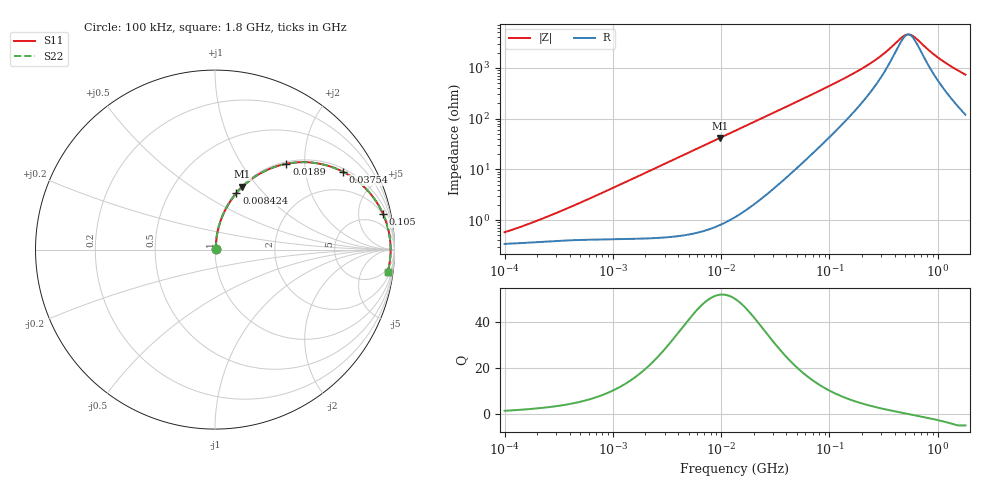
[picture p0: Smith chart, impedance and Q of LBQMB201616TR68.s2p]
! LBQMB201616TR68  S-PARAMETER MODEL  ( General Type )
! Model Generated by TAIYO YUDEN Corporation (http://www.ty-top.com)
! Version 1.0
! TAIYO YUDEN Control No. 191025NI43SB-FBB
! Copyright(c) 2019 TAIYO YUDEN CO.,LTD. All Rights Reserved.
! Product Description (link to TY-COMPAS)
! https://ds.yuden.co.jp/TYCOMPAS/or/detail?pn=LBQMB201616TR68J&u=M
! Products Name : Inductors
! Characteristics :
!  Inductance : 0.68 uH , SRF(min) : 270 MHz , DC Resistance(max) : 0.416 Ohm , Rated Current : 400 mA
!  Case Size : 2.0 x 1.6 / 0.079 x 0.063 [mm/inch] , Thickness : 1.6 / 0.063 [mm/inch]
!  (Conditions: Temperature = 25 degC , DC Bias Current/Voltage = 0A / 0V)
! External Node Assignments :
!  1  o---GGG---o  2
! GND o---------o GND
! Frequency Range : 0.1MHz  -  1800MHz  [ 402 STEP ]
# MHz S RI R 50
! Freq[MHz].  S11 Real  S11 Imag  S21 Real  S21 Imag  S12 Real  S12 Imag  S22 Real  S22 Imag
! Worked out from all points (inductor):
!   401 points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, 100 kHz to 1.8 GHz, reference 50 ohm
!   read as one part in series: L = 702 nH near 259.9 kHz
!   highest Q = 52 at 9.758 MHz (marker M1), where L = 680 nH
!   self-resonance near 535.3 MHz
!   S11 on the Smith chart (normalised r, x): 100 kHz: 1.01, +0.01; 8.424 MHz: 1.01, +0.72; 18.9 MHz: 1.04, +1.62; 37.54 MHz: 1.12, +3.22; 105 MHz: 1.96, +9.24; 1.8 GHz: 3, -15
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0.1  0.00341 0.00464  0.9966 -0.00464  0.9966 -0.00464  0.00341 0.00464
0.19855  0.00377 0.00892  0.9962 -0.00892  0.9962 -0.00892  0.00377 0.00892
0.516129  0.00456 0.0222  0.9954 -0.0222  0.9954 -0.0222  0.00456 0.0222
1.309209  0.00732 0.0554  0.9927 -0.0554  0.9927 -0.0554  0.00732 0.0554
2.66389  0.0171 0.1114  0.9829 -0.1114  0.9829 -0.1114  0.0171 0.1114
5.161158  0.0509 0.2082  0.9491 -0.2082  0.9491 -0.2082  0.0509 0.2082
8.423854  0.1195 0.3147  0.8805 -0.3147  0.8805 -0.3147  0.1195 0.3147
9.75753  0.1529 0.3504  0.8471 -0.3504  0.8471 -0.3504  0.1529 0.3504
13.41641  0.2518 0.4242  0.7482 -0.4242  0.7482 -0.4242  0.2518 0.4242
18.90474  0.3977 0.4781  0.6023 -0.4781  0.6023 -0.4781  0.3977 0.4781
25.99364  0.5519 0.4834  0.4481 -0.4834  0.4481 -0.4834  0.5519 0.4834
37.5353  0.7145 0.433  0.2855 -0.433  0.2855 -0.433  0.7145 0.433
50.36143  0.8129 0.366  0.1871 -0.366  0.1871 -0.366  0.8129 0.366
69.24595  0.8846 0.2875  0.1154 -0.2875  0.1154 -0.2875  0.8846 0.2875
105.0131  0.9371 0.1964  0.0629 -0.1964  0.0629 -0.1964  0.9371 0.1964
218.9722  0.9711 0.0846  0.0289 -0.0846  0.0289 -0.0846  0.9711 0.0846
357.3983  0.9773 0.0347  0.0227 -0.0347  0.0227 -0.0347  0.9773 0.0347
479.5244  0.9784 0.00922  0.0216 -0.00922  0.0216 -0.00922  0.9784 0.00922
555.4434  0.9785 -0.00311  0.0215 0.00311  0.0215 0.00311  0.9785 -0.00311
627.8136  0.9783 -0.0134  0.0217 0.0134  0.0217 0.0134  0.9783 -0.0134
1050.104  0.9747 -0.0606  0.0253 0.0606  0.0253 0.0606  0.9747 -0.0606
1800  0.9619 -0.1262  0.0381 0.1262  0.0381 0.1262  0.9619 -0.1262
